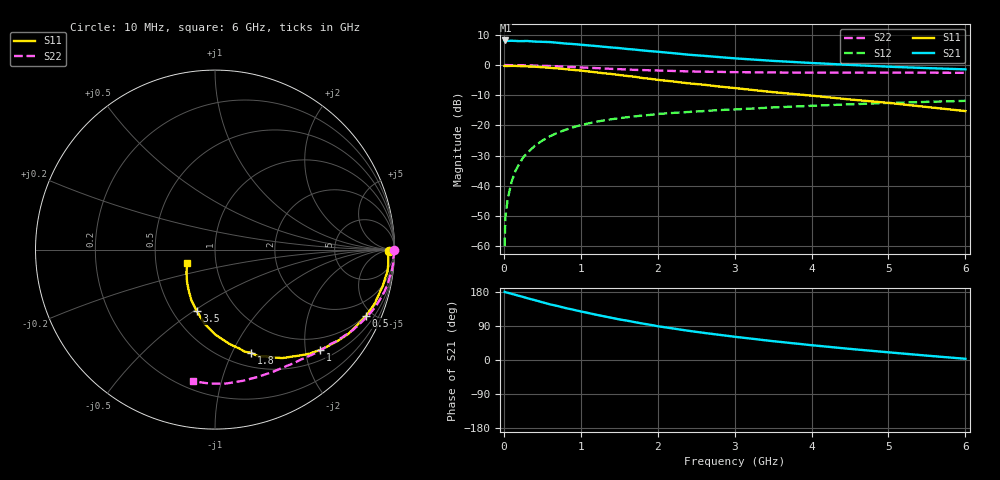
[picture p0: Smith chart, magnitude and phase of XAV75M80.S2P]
! SIEMENS Discrete & RF Semiconductors
! BFY180
! Si NPN RF Bipolar Junction Transistor in MICRO-X
! VCE = 0.75 V  IC = 0.8 mA
! Common Emitter S-Parameters:  May  1997
# GHz  S  MA  R  50
!  f  S11  S21  S12  S22
! GHz  MAG  ANG  MAG  ANG  MAG  ANG  MAG  ANG
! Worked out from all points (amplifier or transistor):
!   36 points, 10 MHz to 6 GHz, reference 50 ohm
!   highest |S21| = 8.1 dB at 20 MHz (marker M1)
!   |S21| within 3 dB of that: start of sweep to 1.693 GHz
!   unconditionally stable (mu >= 1): 3.168 GHz to end of sweep
!   at 250 MHz: K = 0.08, MSG = 19.3 dB, |S12| = -30.6 dB
!   at 1.4 GHz: K = 0.56, MSG = 11.9 dB, |S12| = -18.0 dB
!   at 6 GHz: K = 1.14, MAG = 3.0 dB, |S12| = -11.9 dB
!   S11 on the Smith chart (normalised r, x): 10 MHz: 60, -13; 500 MHz: 0.96, -4.59; 1 GHz: 0.71, -2.31; 1.8 GHz: 0.65, -1.19; 3.5 GHz: 0.66, -0.51; 6 GHz: 0.72, -0.11
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0.01  0.9686 -0.4  2.512 179.7  0.001 92.6  0.9971 -0.2
0.02  0.961 -0.9  2.554 178.9  0.003 91.6  0.9999 -0.6
0.05  0.9653 -2.1  2.508 177.5  0.006 89.6  0.9969 -1.4
0.1  0.9688 -4.7  2.524 174.7  0.0116 86.1  0.9944 -2.9
0.15  0.9689 -7.2  2.508 172.0  0.0176 85.1  0.9958 -4.3
0.25  0.9568 -12.1  2.493 166.5  0.0294 81.9  0.9929 -7.1
0.3  0.9495 -14.1  2.503 163.3  0.0344 79.8  0.9868 -8.4
0.5  0.9198 -23.6  2.425 152.4  0.0561 72.7  0.9728 -13.9
0.6  0.8983 -27.7  2.402 146.8  0.0662 69.9  0.962 -16.4
0.8  0.8559 -36.1  2.27 137.2  0.0844 63.9  0.9393 -21.4
1  0.8104 -43.6  2.172 128.2  0.1009 58.4  0.9133 -25.9
1.1  0.7835 -47.7  2.114 123.9  0.1079 55.9  0.9013 -28.0
1.5  0.6837 -61.5  1.909 107.2  0.1317 47.1  0.8538 -35.8
1.8  0.6098 -70.7  1.748 96.3  0.1458 42.5  0.8262 -40.7
2  0.5682 -76.1  1.661 89.1  0.1546 39.3  0.812 -43.9
2.2  0.5351 -80.8  1.573 83.2  0.1612 36.3  0.798 -47.1
2.4  0.4978 -85.9  1.484 77.1  0.167 34.0  0.7853 -49.9
2.8  0.4407 -94.2  1.354 66.5  0.1797 29.9  0.7701 -55.3
3.5  0.3557 -106.8  1.172 49.7  0.1985 23.6  0.7536 -64.6
4.5  0.269 -123.2  1.006 29.3  0.2239 14.8  0.7472 -78.1
5.5  0.2019 -141.9  0.89 11.5  0.2458 6.3  0.747 -92.3
6  0.1728 -153.9  0.848 3.2  0.2554 1.7  0.7436 -99.5
